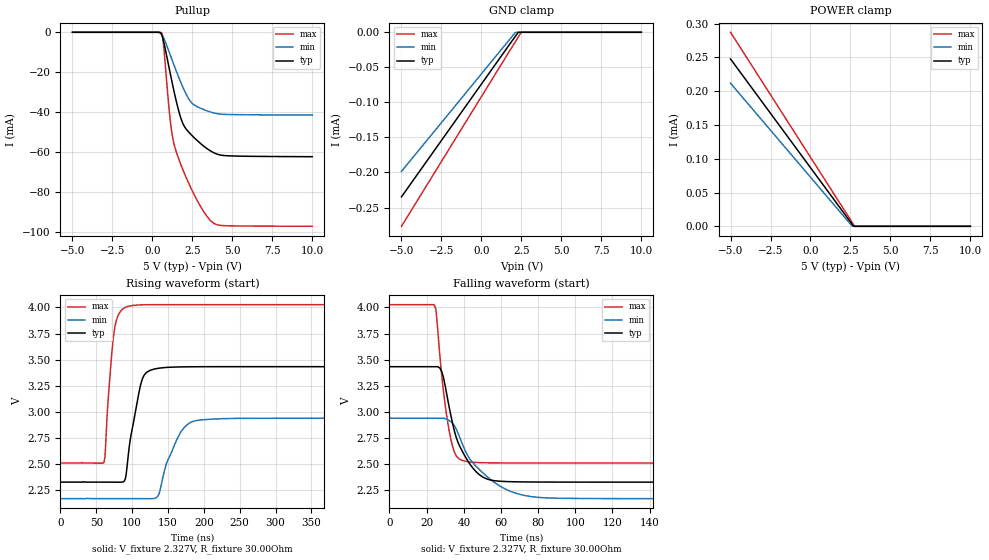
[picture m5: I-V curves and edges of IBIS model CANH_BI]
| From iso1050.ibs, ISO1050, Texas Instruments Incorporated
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|   CANH Model
[Model]   CANH_BI
Model_type   I/O_open_source
| Signals   CANH
Vinh = 0.9V
Vinl = 0.5V
Rref = 30   |Note: 60 Ohm differential load;
Vref = 2.327V   |tr and tf measured single-ended
Vmeas = 2.3V
| variable   typ   min   max
C_comp   8.9236pF   9.3146pF   8.5841pF
|   typ   min   max
[Temperature Range]   40   125   -55
[Voltage Range]   5.0V   4.75V   5.25V
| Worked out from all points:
|   slope of the pullup table from 0 to 0.75 V, typ, clamps not added: 119 ohm
|   rising waveform, V_fixture 2.327V, R_fixture 30.00Ohm: 20-80 % time 16.3ns typ, 24.8ns min, 10ns max; typ from 2.33 V to 3.43 V
|   falling waveform, V_fixture 2.327V, R_fixture 30.00Ohm: 20-80 % time 11.2ns typ, 19.5ns min, 5.93ns max; typ from 3.43 V to 2.33 V
[GND Clamp]
|   Voltage   I(typ)   I(min)   I(max)
-5V       -234.7uA   -198.4uA   -276.8uA
2.085V    -6.935uA   -1.2uA     -14.84uA
2.312V    0A         0A         -6.47uA
2.462V    0A         0A         -892.6nA
2.538V    0A         0A         0A
10V       0A         0A         0A
[Pullup]
|   Voltage   I(typ)   I(min)   I(max)
-5V       0A         100pA      100pA
577.9mV   -1.147mA   -945.5uA   -274.4uA
653.3mV   -3.012mA   -1.947mA   -2.661mA
728.6mV   -5.522mA   -3.244mA   -8.5mA
1.106V    -20.2mA    -11.13mA   -43.34mA
1.256V    -26mA      -14.4mA    -52.37mA
1.407V    -31.51mA   -17.62mA   -57.57mA
1.709V    -41.12mA   -23.77mA   -64.71mA
2.01V     -47.28mA   -29.31mA   -70.77mA
2.538V    -52.17mA   -35.91mA   -80.06mA
3.744V    -59.89mA   -40.16mA   -95.03mA
10V       -62.28mA   -41.46mA   -97.12mA
[POWER Clamp]
|   Voltage   I(typ)   I(min)   I(max)
-5V       247.7uA    211.9uA    287.3uA
2.613V    2.766uA    92.82nA    5.567uA
2.688V    340.9nA    0A         2.779uA
2.764V    0A         0A         0A
10V       0A         0A         0A
[Ramp]
R_load = 30.00Ohm
|   typ   min   max
dV/dt_r   663.537mV/16.275ns  462.522mV/24.794ns  910.178mV/10.035ns
dV/dt_f   663.537mV/11.194ns  462.522mV/19.463ns  910.178mV/5.932ns
[Rising Waveform]
V_fixture = 2.327V
V_fixture_min = 2.169V
V_fixture_max = 2.510V
R_fixture = 30.00Ohm
|   Time   V(typ)   V(min)   V(max)
0s        2.327V     2.169V     2.51V
61ns      2.327V     2.169V     2.523V
75ns      2.327V     2.169V     3.775V
91ns      2.373V     2.169V     4.003V
112ns     3.264V     2.169V     4.025V
126ns     3.4V       2.169V     4.027V
137ns     3.418V     2.206V     4.027V
164ns     3.43V      2.759V     4.027V
184ns     3.432V     2.907V     4.027V
500ns     3.433V     2.94V      4.027V
[Falling Waveform]
V_fixture = 2.327V
V_fixture_min = 2.169V
V_fixture_max = 2.510V
R_fixture = 30.00Ohm
|   Time   V(typ)   V(min)   V(max)
0s        3.433V     2.94V      4.027V
24ns      3.433V     2.94V      4.027V
25ns      3.433V     2.94V      3.983V
28ns      3.391V     2.94V      3.368V
33ns      2.968V     2.906V     2.739V
36ns      2.751V     2.833V     2.576V
42ns      2.535V     2.585V     2.524V
54ns      2.349V     2.358V     2.512V
84ns      2.328V     2.177V     2.51V
500ns     2.327V     2.169V     2.51V
